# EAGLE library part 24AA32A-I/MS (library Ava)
IC EEPROM 32KBIT 400KHZ
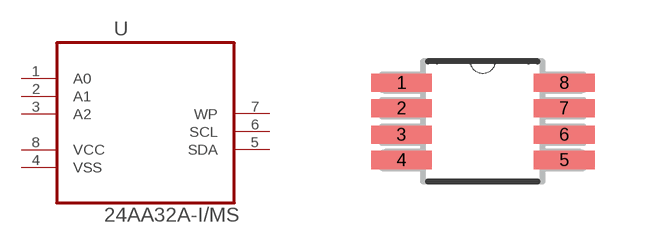
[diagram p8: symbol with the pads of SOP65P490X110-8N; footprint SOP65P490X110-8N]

Designator prefix U

## 24AA32A-I/MS (MPN: 24AA32A-I/MS; OC_FARNELL: 1331296; OC_NEWARK: 40C2562; PACKAGE: MSOP8; SUPPLIER: Microchip)  [SOP65P490X110-8N]
1  A0  nc
2  A1  nc
3  A2  nc
4  VSS  pas
5  SDA
6  SCL  in
7  WP  in
8  VCC  pwr

## Footprint SOP65P490X110-8N (pad centres in mm)
smd 1.524 x 0.457: 1 -2.032,0.965; 2 -2.032,0.33; 3 -2.032,-0.33; 4 -2.032,-0.965; 5 2.032,-0.965; 6 2.032,-0.33; 7 2.032,0.33; 8 2.032,0.965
